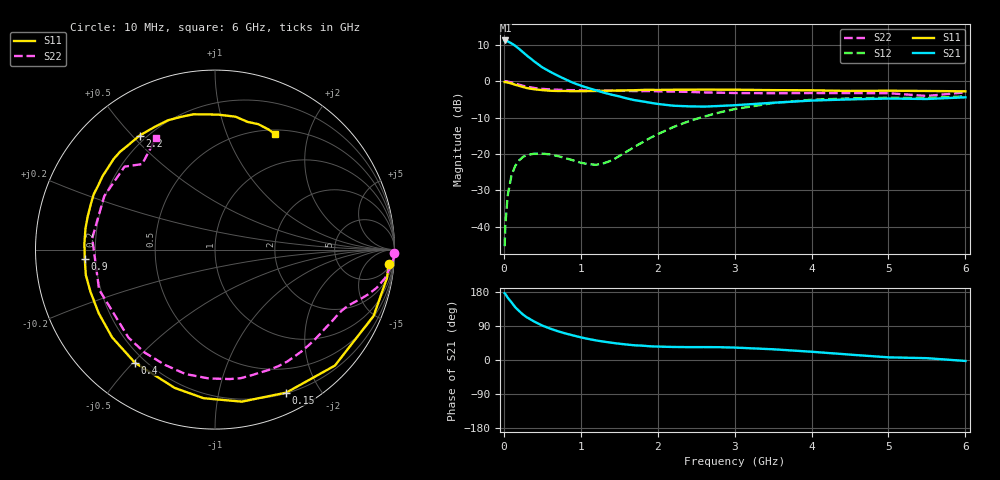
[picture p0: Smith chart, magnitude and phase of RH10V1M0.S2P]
! SIEMENS Small Signal Semiconductors
! BFR106
! Si NPN RF Bipolar Junction Transistor in SOT23
! VCE = 10 V  IC = 1 mA
! Common Emitter S-Parameters:  August  1996
# GHz  S  MA  R  50
!  f  S11  S21  S12  S22
! GHz  MAG  ANG  MAG  ANG  MAG  ANG  MAG  ANG
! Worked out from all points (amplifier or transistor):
!   36 points, 10 MHz to 6 GHz, reference 50 ohm
!   highest |S21| = 11.2 dB at 20 MHz (marker M1)
!   |S21| within 3 dB of that: start of sweep to 235.9 MHz
!   unconditionally stable (mu >= 1): 865.7 MHz to 1.837 GHz; 3.219 GHz to end of sweep
!   at 250 MHz: K = 0.25, MSG = 14.4 dB, |S12| = -20.8 dB
!   at 1.4 GHz: K = 1.39, MAG = 5.3 dB, |S12| = -21.8 dB
!   at 6 GHz: K = 1.02, MAG = -0.9 dB, |S12| = -4.2 dB
!   S11 on the Smith chart (normalised r, x): 10 MHz: 8, -22; 150 MHz: 0.21, -1.60; 400 MHz: 0.16, -0.51; 900 MHz: 0.16, -0.03; 2.2 GHz: 0.17, +0.52; 6 GHz: 0.55, +1.50
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0.01  0.9715 -4.7  3.607 176.3  0.0054 88.7  0.9999 -1.2
0.02  0.9711 -9.4  3.626 174.1  0.0108 82.8  0.9999 -2.2
0.05  0.958 -22.6  3.526 164.7  0.0268 76.8  0.9865 -5.0
0.1  0.9296 -44.0  3.304 152.0  0.0511 66.0  0.9602 -9.6
0.15  0.8902 -63.5  3.053 138.8  0.069 55.2  0.9256 -13.3
0.2  0.8601 -80.0  2.766 129.0  0.0818 47.5  0.8928 -16.0
0.25  0.8304 -94.4  2.493 119.7  0.0913 40.4  0.8632 -18.2
0.3  0.8028 -106.2  2.245 112.6  0.0964 35.6  0.8388 -20.0
0.4  0.772 -125.3  1.854 100.9  0.101 27.6  0.8038 -22.9
0.5  0.7535 -139.5  1.549 90.9  0.1012 22.6  0.7831 -25.8
0.6  0.7386 -151.3  1.351 83.0  0.0984 19.9  0.7714 -28.8
0.9  0.7274 -176.0  0.951 64.9  0.0817 22.8  0.751 -38.5
1.1  0.7312 170.7  0.803 55.5  0.0724 35.0  0.7459 -45.8
1.3  0.7364 160.2  0.695 48.4  0.0745 54.2  0.7423 -53.4
1.6  0.7483 146.8  0.579 40.7  0.108 75.7  0.7349 -65.5
2.2  0.7616 123.5  0.46 34.4  0.233 78.4  0.7186 -92.9
2.8  0.7635 104.4  0.456 33.8  0.3707 64.6  0.6947 -124.3
3.5  0.7525 88.8  0.505 28.3  0.5005 45.5  0.683 -161.0
4.5  0.7342 75.6  0.562 14.2  0.5796 21.2  0.6852 154.2
5  0.7393 71.0  0.577 7.0  0.5918 12.1  0.6837 137.5
5.5  0.7327 65.9  0.569 4.8  0.5861 7.6  0.6258 130.4
6  0.7252 62.6  0.6 -2.5  0.6183 -0.7  0.7025 118.0
